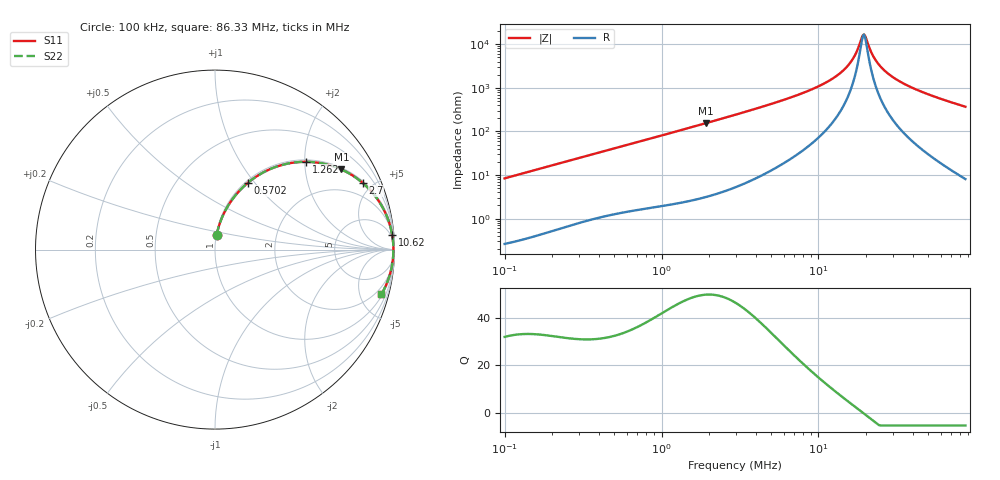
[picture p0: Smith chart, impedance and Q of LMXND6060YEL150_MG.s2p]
! LMXND6060YEL150_MG  S-PARAMETER MODEL  ( General Type )
! Model Generated by TAIYO YUDEN Corporation (http://www.ty-top.com)
! Version 1.0
! TAIYO YUDEN Control No. 191025NI43SB-FBB
! Copyright(c) 2019 TAIYO YUDEN CO.,LTD. All Rights Reserved.
! Product Description (link to TY-COMPAS)
! https://ds.yuden.co.jp/TYCOMPAS/or/detail?pn=LMXND6060YEL150MMG&u=M
! Products Name : Inductors
! Characteristics :
!  Inductance : 15 uH , SRF(min) : 10 MHz , DC Resistance(max) : 0.091 Ohm
!  Rated Current : Saturation :2500 mA , Temp Rise : 1900 mA
!  Case Size : 6.0 x 6.0 / 0.236 x 0.236 [mm/inch] , Thickness : 4.5 / 0.177 [mm/inch]
!  (Conditions: Temperature = 25 degC , DC Bias Current/Voltage = 0A / 0V)
! External Node Assignments :
!  1  o---GGG---o  2
! GND o---------o GND
! Frequency Range : 0.1MHz  -  86.325287MHz  [ 402 STEP ]
# MHz S RI R 50
! Freq[MHz].  S11 Real  S11 Imag  S21 Real  S21 Imag  S12 Real  S12 Imag  S22 Real  S22 Imag
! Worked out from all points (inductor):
!   401 points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, 100 kHz to 86.33 MHz, reference 50 ohm
!   read as one part in series: L = 13.3 uH near 103.4 kHz
!   highest Q = 49.5 at 1.926 MHz (marker M1), where L = 12.9 uH
!   self-resonance near 19.18 MHz
!   S11 on the Smith chart (normalised r, x): 100 kHz: 1.01, +0.17; 570.2 kHz: 1.03, +0.93; 1.262 MHz: 1.04, +2.03; 2.7 MHz: 1.09, +4.40; 10.62 MHz: 3, +24; 86.33 MHz: 1.16, -7.37
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0.1  0.00954 0.0828  0.9905 -0.0828  0.9905 -0.0828  0.00954 0.0828
0.310315  0.0681 0.2362  0.9319 -0.2362  0.9319 -0.2362  0.0681 0.2362
0.570237  0.1838 0.3727  0.8162 -0.3727  0.8162 -0.3727  0.1838 0.3727
0.962956  0.3788 0.4731  0.6212 -0.4731  0.6212 -0.4731  0.3788 0.4731
1.261978  0.5078 0.4891  0.4922 -0.4891  0.4922 -0.4891  0.5078 0.4891
1.925575  0.7038 0.4466  0.2962 -0.4466  0.2962 -0.4466  0.7038 0.4466
2.700022  0.8236 0.3708  0.1764 -0.3708  0.1764 -0.3708  0.8236 0.3708
2.938117  0.847 0.3494  0.153 -0.3494  0.153 -0.3494  0.847 0.3494
5.584729  0.9535 0.1949  0.0465 -0.1949  0.0465 -0.1949  0.9535 0.1949
9.117424  0.9827 0.1047  0.0173 -0.1047  0.0173 -0.1047  0.9827 0.1047
10.61537  0.9872 0.0813  0.0128 -0.0813  0.0128 -0.0813  0.9872 0.0813
13.22391  0.9915 0.0502  0.00854 -0.0502  0.00854 -0.0502  0.9915 0.0502
15.39653  0.9931 0.03  0.00686 -0.03  0.00686 -0.03  0.9931 0.03
16.75423  0.9937 0.0191  0.00631 -0.0191  0.00631 -0.0191  0.9937 0.0191
18.85849  0.9941 0.00393  0.00594 -0.00393  0.00594 -0.00393  0.9941 0.00393
19.50687  0.9941 -0.000371  0.00592 0.000371  0.00592 0.000371  0.9941 -0.000371
20.17755  0.9941 -0.00467  0.00593 0.00467  0.00593 0.00467  0.9941 -0.00467
21.58886  0.9939 -0.0133  0.00608 0.0133  0.00608 0.0133  0.9939 -0.0133
23.09889  0.9936 -0.022  0.00638 0.022  0.00638 0.022  0.9936 -0.022
28.29276  0.9917 -0.0487  0.00827 0.0487  0.00827 0.0487  0.9917 -0.0487
43.17018  0.9815 -0.1112  0.0185 0.1112  0.0185 0.1112  0.9815 -0.1112
86.32529  0.9267 -0.25  0.0733 0.25  0.0733 0.25  0.9267 -0.25
